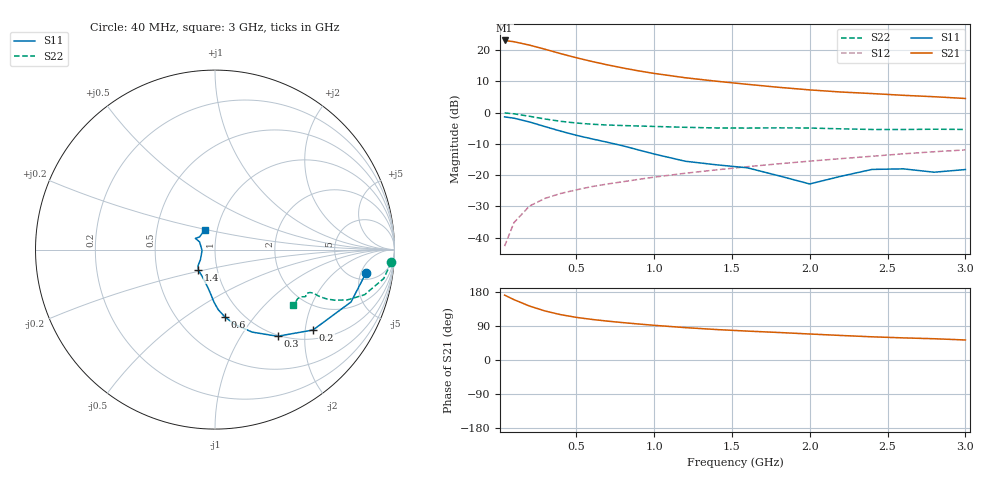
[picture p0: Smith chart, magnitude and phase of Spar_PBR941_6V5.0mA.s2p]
! Filename:  PBR941M.S2P  Version:  3.0
! NXP part #:  PBR941  Date: July 1998
! Bias condition:  Vce=6V, Ic=5.0mA
#  MHz  S  MA  R 50
! Freq  S11  S21  S12  S22
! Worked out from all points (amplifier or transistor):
!   21 points, 40 MHz to 3 GHz, reference 50 ohm
!   highest |S21| = 23.0 dB at 40 MHz (marker M1)
!   |S21| within 3 dB of that: start of sweep to 313.4 MHz
!   unconditionally stable (mu >= 1): 1.323 GHz to 2.52 GHz
!   at 300 MHz: K = 0.48, MSG = 23.8 dB, |S12| = -27.4 dB
!   at 1 GHz: K = 0.94, MSG = 16.6 dB, |S12| = -20.7 dB
!   at 3 GHz: K = 0.99, MSG = 8.2 dB, |S12| = -11.9 dB
!   lowest NFmin = 1.34 dB at 900 MHz
!   S11 on the Smith chart (normalised r, x): 40 MHz: 6.60, -6.20; 200 MHz: 1.23, -2.20; 300 MHz: 0.98, -1.47; 600 MHz: 0.83, -0.73; 1.4 GHz: 0.81, -0.19; 3 GHz: 0.87, +0.19
40  0.8518 -8.7  14.18 171.2  0.007316 83.6  0.9852 -4.1
100  0.8122 -21.1  13.53 159.3  0.0174 80.2  0.9537 -9.7
200  0.7064 -39.4  11.95 142.3  0.03207 71.4  0.8705 -16.8
300  0.5955 -54.2  10.26 129.3  0.0425 67.6  0.7878 -20.9
400  0.5041 -65.8  8.731 119.7  0.05085 65.8  0.7241 -22.9
500  0.4329 -75.0  7.519 112.5  0.05801 65.7  0.6799 -23.8
600  0.3798 -81.6  6.553 107.1  0.06546 66.4  0.6506 -24.1
700  0.3348 -87.0  5.781 102.6  0.07205 67.2  0.6318 -24.1
800  0.2936 -91.0  5.149 98.6  0.07829 68.2  0.6195 -24.0
900  0.2524 -95.1  4.633 95.0  0.0854 69.3  0.609 -23.9
1000  0.2174 -100.2  4.219 91.6  0.09273 70.2  0.5995 -23.9
1200  0.1666 -115.1  3.596 85.5  0.1071 71.3  0.5804 -24.3
1400  0.1461 -129.5  3.165 80.4  0.1212 72.2  0.5663 -25.4
1600  0.1307 -136.3  2.823 76.3  0.1364 73.4  0.5647 -26.5
1800  0.09772 -145.9  2.529 72.6  0.1514 74.3  0.5692 -27.2
2000  0.07218 -176.0  2.299 68.6  0.1671 74.4  0.565 -27.7
2200  0.0957 153.7  2.127 64.7  0.1832 74.3  0.5491 -28.6
2400  0.1232 150.3  2.009 61.2  0.2 74.4  0.5358 -30.6
2600  0.1259 150.4  1.885 58.4  0.2187 74.6  0.5354 -33.1
2800  0.1112 140.4  1.788 56.1  0.2363 74.6  0.5409 -34.9
3000  0.1227 118.3  1.677 52.8  0.2528 74.0  0.5363 -35.4
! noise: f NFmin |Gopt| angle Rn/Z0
500  1.372  0.368  12.68  0.302
900  1.344  0.322  23.15  0.263
1000  1.403  0.31  28.56  0.283
2000  2.036  0.07  103.2  0.226
